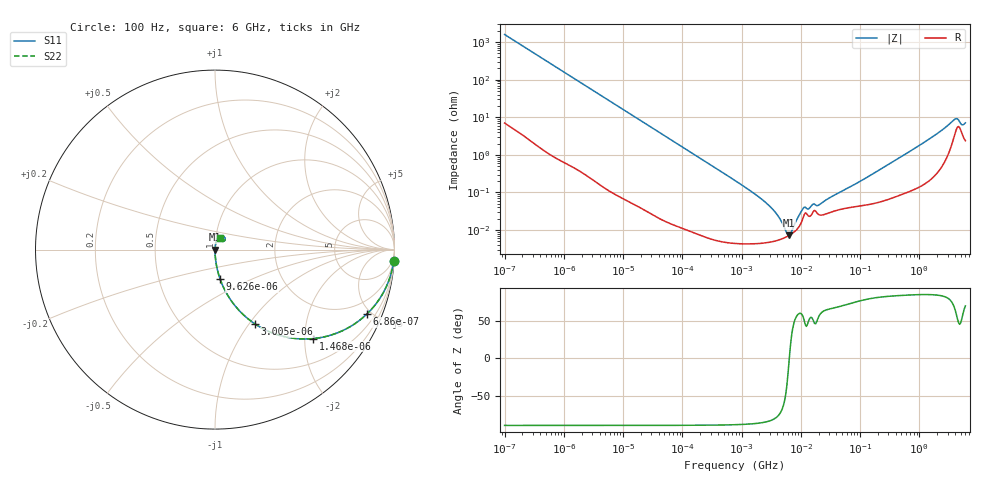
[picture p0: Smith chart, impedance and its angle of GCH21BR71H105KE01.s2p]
!Murata Part Number: GCH21BR71H105KE01
!These Parameters are Measured in Series Mode Connection
!Data Generated on Jun 19, 2026
!  o--ll--o
!Port1  Port2
!  o------o
!Operation Temp=25[degC], DC Bias Voltage=0[V]
!Freq. Start=100[Hz] Stop=6[GHz] 401[Steps]
# Hz S RI R 50
!Freq.(Hz) S11(Real) S11(Imag) S21(Real) S21(Imag) S12(Real) S12(Imag) S22(Real) S22(Imag)
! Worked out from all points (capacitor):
!   401 points, 100 Hz to 6 GHz, reference 50 ohm
!   read as one part in series: C = 995 nF near 109 Hz
!   lowest |Z| = 7.21 mohm at 6.353 MHz (marker M1)
!   series resonance near 6.388 MHz, so ESL is about 620 pH
!   S11 on the Smith chart (normalised r, x): 100 Hz: 1, -32; 686 Hz: 1.02, -4.68; 1.468 kHz: 1.01, -2.19; 3.005 kHz: 1.00, -1.07; 9.626 kHz: 1.00, -0.34; 6 GHz: 1.05, +0.13
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100  0.9958 -0.0623  0.00418 0.0623  0.00418 0.0623  0.9958 -0.0623
335  0.9574 -0.2  0.0426 0.2  0.0426 0.2  0.9574 -0.2
686  0.8446 -0.3604  0.1554 0.3604  0.1554 0.3604  0.8446 -0.3604
1468  0.545 -0.4959  0.455 0.4959  0.455 0.4959  0.545 -0.4959
2008  0.3914 -0.4859  0.6086 0.4859  0.6086 0.4859  0.3914 -0.4859
3005  0.2242 -0.415  0.7758 0.415  0.7758 0.415  0.2242 -0.415
5143  0.0905 -0.2849  0.9095 0.2849  0.9095 0.2849  0.0905 -0.2849
9626  0.028 -0.163  0.972 0.163  0.972 0.163  0.028 -0.163
40335  0.00182 -0.0401  0.9982 0.0401  0.9982 0.0401  0.00182 -0.0401
774597  4.82e-05 -0.00208  1 0.00208  1 0.00208  4.82e-05 -0.00208
2713602  4.65e-05 -0.000494  1 0.000494  1 0.000494  4.65e-05 -0.000494
3882480  5.21e-05 -0.000266  0.9999 0.000266  0.9999 0.000266  5.21e-05 -0.000266
5554849  6.43e-05 -7.25e-05  0.9999 7.25e-05  0.9999 7.25e-05  6.43e-05 -7.25e-05
6353432  7.2e-05 -2.8e-06  0.9999 2.8e-06  0.9999 2.8e-06  7.2e-05 -2.8e-06
7266822  8.27e-05 6.79e-05  0.9999 -6.79e-05  0.9999 -6.79e-05  8.27e-05 6.79e-05
1.087309e7  0.000205 0.000309  0.9998 -0.000309  0.9998 -0.000309  0.000205 0.000309
1.555665e7  0.000274 0.000378  0.9997 -0.000378  0.9997 -0.000378  0.000274 0.000378
2.035112e7  0.000254 0.000392  0.9997 -0.000392  0.9997 -0.000392  0.000254 0.000392
3.124326e8  0.000699 0.00572  0.9993 -0.00572  0.9993 -0.00572  0.000699 0.00572
1.565993e9  0.003 0.028  0.997 -0.028  0.997 -0.028  0.003 0.028
3.8344e9  0.0339 0.0749  0.9661 -0.0749  0.9661 -0.0749  0.0339 0.0749
6e9  0.0274 0.0637  0.9726 -0.0637  0.9726 -0.0637  0.0274 0.0637
